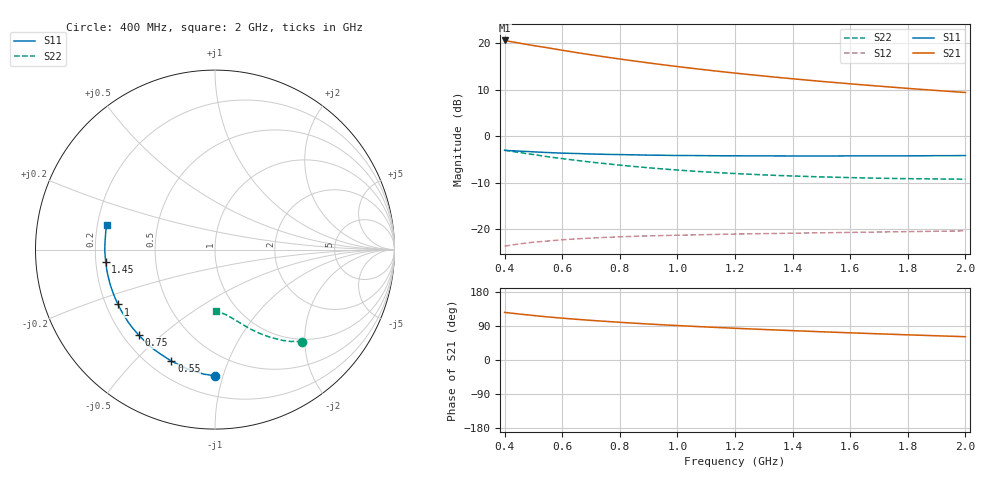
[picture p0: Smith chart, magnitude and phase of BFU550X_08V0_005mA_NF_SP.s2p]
! Filename:  P:\Prog\Test\Noise\ATS_data\Testdata_Net\BFU550X no attenuator noise\BFU550X_APG2013_44_C05_08p0V_005mA_NF_CM01_D.sf
! Date/Time: Fri 26/Jul/2013 14:37:13
! BFU550X_APG2013_44_C05_08p0V_1to10mA_NF_CM01_Bias4_R.sf
! Noise Parameter Data File
! BFU550X_APG2013_44_C05_08p0V_1to10mA_NF_CM01
! Date/time: Wed Jul 24 17:16:38 2013
! VAR V_out= 8.000000
! VAR I_out= 5.000000
! VAR V_in= 0.805900
! VAR I_in= 0.053110
! Device data file deembeded for feedlines and parallel
! Original file: \BFU550X no attenuator noise\BFU550X_APG2013_44_C05_08p0V_005mA_NF_CM01_R.sf
! Feed-files: PR005V01_100713_Feed1.s2p, PR005V01_100713_Feed2.s2p
! Parallel-file: PR005V01_100713_Par.s2p
# MHz S MA R 50
!  Freq-MHz  S11-mag  S11-arg  S21-mag  S21-arg  S12-mag  S12-arg  S22-mag  S22-arg
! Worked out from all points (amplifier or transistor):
!   37 points, 400 MHz to 2 GHz, reference 50 ohm
!   highest |S21| = 20.6 dB at 400 MHz (marker M1)
!   |S21| within 3 dB of that: start of sweep to 690.9 MHz
!   unconditionally stable (mu >= 1): nowhere
!   at 500 MHz: K = 0.26, MSG = 21.2 dB, |S12| = -22.8 dB
!   at 1.1 GHz: K = 0.55, MSG = 17.7 dB, |S12| = -21.2 dB
!   at 2 GHz: K = 0.89, MSG = 14.9 dB, |S12| = -20.4 dB
!   lowest NFmin = 0.65 dB at 460 MHz
!   S11 on the Smith chart (normalised r, x): 400 MHz: 0.34, -0.94; 550 MHz: 0.29, -0.64; 750 MHz: 0.26, -0.42; 1 GHz: 0.25, -0.25; 1.45 GHz: 0.24, -0.05; 2 GHz: 0.24, +0.11
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400  0.7052 -90.0  10.73 125.7  0.06554 47.0  0.7067 -46.5
420  0.6985 -93.0  10.44 123.9  0.06701 45.9  0.6892 -48.0
440  0.6943 -96.2  10.2 122.2  0.06859 44.7  0.6759 -49.2
460  0.6883 -99.0  9.93 120.6  0.06987 43.5  0.6624 -50.6
500  0.6785 -104.7  9.461 117.4  0.07227 41.6  0.6352 -53.0
550  0.667 -111.3  8.937 113.7  0.07447 39.4  0.6013 -55.7
600  0.6572 -117.0  8.419 110.4  0.07672 37.5  0.574 -58.0
650  0.6511 -122.3  7.94 107.4  0.07861 35.9  0.5494 -60.2
700  0.6434 -127.4  7.519 104.5  0.08004 34.5  0.5263 -62.2
750  0.6381 -131.8  7.123 102.0  0.08149 33.4  0.5069 -63.9
800  0.6341 -136.1  6.775 99.5  0.08262 32.3  0.4883 -65.6
850  0.6303 -140.1  6.448 97.2  0.08368 31.4  0.4722 -67.1
900  0.6258 -143.9  6.149 94.9  0.08452 30.6  0.4575 -68.5
950  0.6233 -147.3  5.873 92.8  0.08529 29.9  0.444 -69.9
1000  0.6203 -150.5  5.617 90.9  0.08599 29.4  0.4324 -71.1
1100  0.6172 -156.4  5.165 87.2  0.08728 28.6  0.4121 -73.4
1200  0.6155 -161.8  4.78 83.7  0.08846 27.9  0.3963 -75.5
1300  0.614 -166.7  4.445 80.5  0.08946 27.6  0.3837 -77.5
1450  0.6128 -173.4  4.017 76.0  0.09086 27.3  0.3688 -80.3
1500  0.6131 -175.5  3.889 74.5  0.09128 27.3  0.3646 -81.2
1750  0.6145 175.2  3.362 67.7  0.09346 27.6  0.351 -85.5
2000  0.6191 167.0  2.956 61.5  0.0959 28.5  0.3448 -89.5
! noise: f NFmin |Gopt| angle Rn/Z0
400  0.7029  0.18  42.87  0.1073
460  0.6517  0.1416  60.58  0.091
600  0.7049  0.1741  68.86  0.1046
800  0.7261  0.189  86.09  0.0938
1000  0.7695  0.217  102.9  0.0858
1200  0.8108  0.2567  117.8  0.0788
1400  0.8382  0.2929  128.9  0.0746
1600  0.8505  0.3218  143.9  0.0621
1800  0.8877  0.3557  154.8  0.0548
2000  0.9363  0.3871  169.9  0.0474
